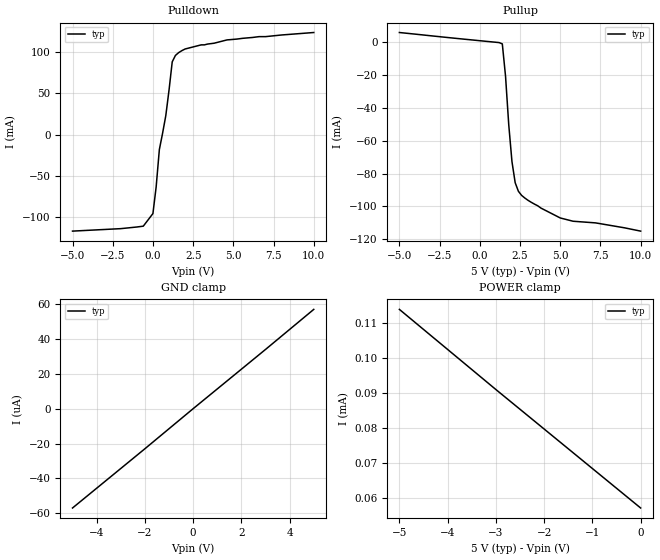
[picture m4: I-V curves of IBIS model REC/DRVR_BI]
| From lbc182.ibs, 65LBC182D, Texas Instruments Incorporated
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|   Driver Output  MODEL
[Model]   REC/DRVR_BI
Model_type   I/O
| Signals   A,B
Vinl = 2.1V
Vinh = 2.5V
Vmeas = 2.3V   |Reference voltage for timing measurements
Cref = 5pF   |Timing specification test load capacitance value
Rref = 54   |Note: 54 Ohm load; single-ended configuration
| variable   typ   min   max
C_comp   1.0pF   NA   NA
|   typ   min   max
[Temperature Range]   25.0   NA   NA
[Voltage range]   5.0V   4.75V   5.25V
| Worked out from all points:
|   slope of the pulldown table from 0 to 0.75 V, typ, clamps not added: 6.61 ohm
|   slope of the pullup table from 0 to 0.75 V, typ, clamps not added: 1.05 kohm
[Pulldown]
|   Voltage   I(typ)   I(min)   I(max)
-5V       -117mA     NA         NA
-600mV    -111mA     NA         NA
0V        -95.7mA    NA         NA
200mV     -63.5mA    NA         NA
400mV     -18mA      NA         NA
800mV     23.1mA     NA         NA
1.2V      88.4mA     NA         NA
1.4V      96.2mA     NA         NA
1.6V      99.6mA     NA         NA
2V        104mA      NA         NA
4.6V      115mA      NA         NA
10V       124mA      NA         NA
[Pullup]
|   Voltage   I(typ)   I(min)   I(max)
| Note that the[Pullup]voltage table is referenced to Vcc
| and is calculated using Vtable=Vcc - Vmeasured.
-5V       5.64mA     NA         NA
1.4V      -1.28mA    NA         NA
1.6V      -20.9mA    NA         NA
1.8V      -50.4mA    NA         NA
2V        -72.8mA    NA         NA
2.2V      -85.6mA    NA         NA
2.4V      -90.8mA    NA         NA
3V        -96.3mA    NA         NA
5V        -107mA     NA         NA
5.8V      -109mA     NA         NA
7.2V      -110mA     NA         NA
10V       -115mA     NA         NA
[GND_clamp]
|   Voltage   I(typ)   I(min)   I(max)
| Outputs in High Impedance (off)
-5V       -57uA      NA         NA
-2V       -23uA      NA         NA
0V        0A         NA         NA
3V        34uA       NA         NA
5V        57uA       NA         NA
[POWER_clamp]
|   Voltage   I(typ)   I(min)   I(max)
| Note that the [POWER_clamp] voltage table is referenced to Vcc
| and is calculated using Vtable = Vcc - Vmeasured.
| Outputs in Tri-state.
-5V       114uA      NA         NA
-3V       91uA       NA         NA
0V        57uA       NA         NA
[Ramp]
|   typ   min   max
dV/dt_r   1.248/506ns   NA   NA
dV/dt_f   1.266/573ns   NA   NA
R_load = 54ohm | Note: The measurement is on a differential configuration
